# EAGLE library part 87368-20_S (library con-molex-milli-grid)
RECEPTACAL
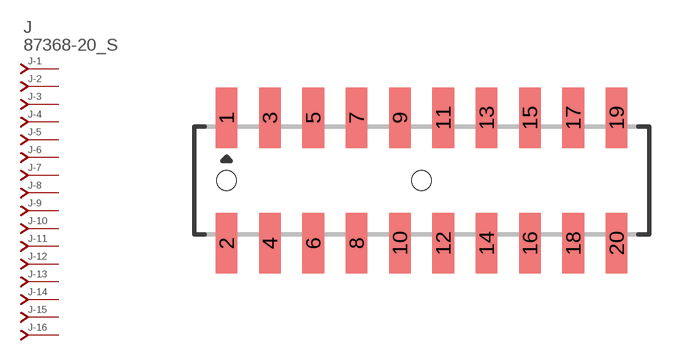
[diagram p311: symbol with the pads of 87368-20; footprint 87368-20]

Designator prefix J; gates -1=J-NV -2=J-N -3=J-N -4=J-N -5=J-N -6=J-N -7=J-N -8=J-N -9=J-N -10=J-N -11=J-N -12=J-N -13=J-N -14=J-N -15=J-N -16=J-N -17=J-N -18=J-N -19=J-N -20=J-N

## 87368-20_S  [87368-20]
1  -1:J  pas
2  -2:J  pas
3  -3:J  pas
4  -4:J  pas
5  -5:J  pas
6  -6:J  pas
7  -7:J  pas
8  -8:J  pas
9  -9:J  pas
10  -10:J  pas
11  -11:J  pas
12  -12:J  pas
13  -13:J  pas
14  -14:J  pas
15  -15:J  pas
16  -16:J  pas
17  -17:J  pas
18  -18:J  pas
19  -19:J  pas
20  -20:J  pas

## Footprint 87368-20 (pad centres in mm)
RECEPTACAL SMD Dual Row, Side Entry
smd 1 x 2.8: 1 -9,2.9; 2 -9,-2.9; 3 -7,2.9; 4 -7,-2.9; 5 -5,2.9; 6 -5,-2.9; 7 -3,2.9; 8 -3,-2.9; 9 -1,2.9; 10 -1,-2.9; 11 1,2.9; 12 1,-2.9; 13 3,2.9; 14 3,-2.9; 15 5,2.9; 16 5,-2.9; 17 7,2.9; 18 7,-2.9; 19 9,2.9; 20 9,-2.9
hole 0.914 at -9,0
hole 0.914 at 0,0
